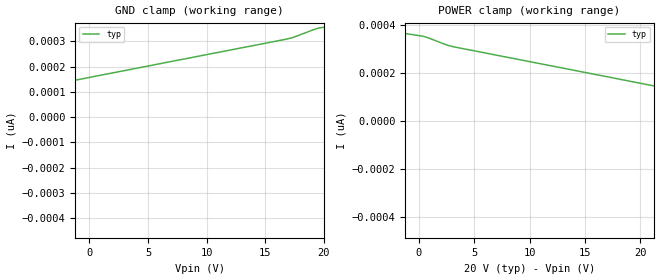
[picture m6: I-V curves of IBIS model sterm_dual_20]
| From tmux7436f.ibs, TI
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| sterm_dual_20
[Model]   sterm_dual_20
Model_type   Terminator
|   typ   min   max
C_comp   4.014581e-12   NA   NA
[Voltage Range]   20   NA   NA
[Temperature Range]   27   NA   NA
[Power Clamp Reference]   20   NA   NA
[GND Clamp Reference]   0   NA   NA
[GND Clamp]
|   Voltage   I(typ)   I(min)   I(max)
-25V      -63.89uA   NA         NA
-20V      -10.3nA    NA         NA
-19.55V   -22.3pA    NA         NA
16.82V    309pA      NA         NA
19.55V    352.8pA    NA         NA
20V       356pA      NA         NA
[POWER Clamp]
|   Voltage   I(typ)   I(min)   I(max)
-5V       391.3pA    NA         NA
454.5mV   352.8pA    NA         NA
3.182V    309pA      NA         NA
39.55V    -22.3pA    NA         NA
40V       -10.3nA    NA         NA
